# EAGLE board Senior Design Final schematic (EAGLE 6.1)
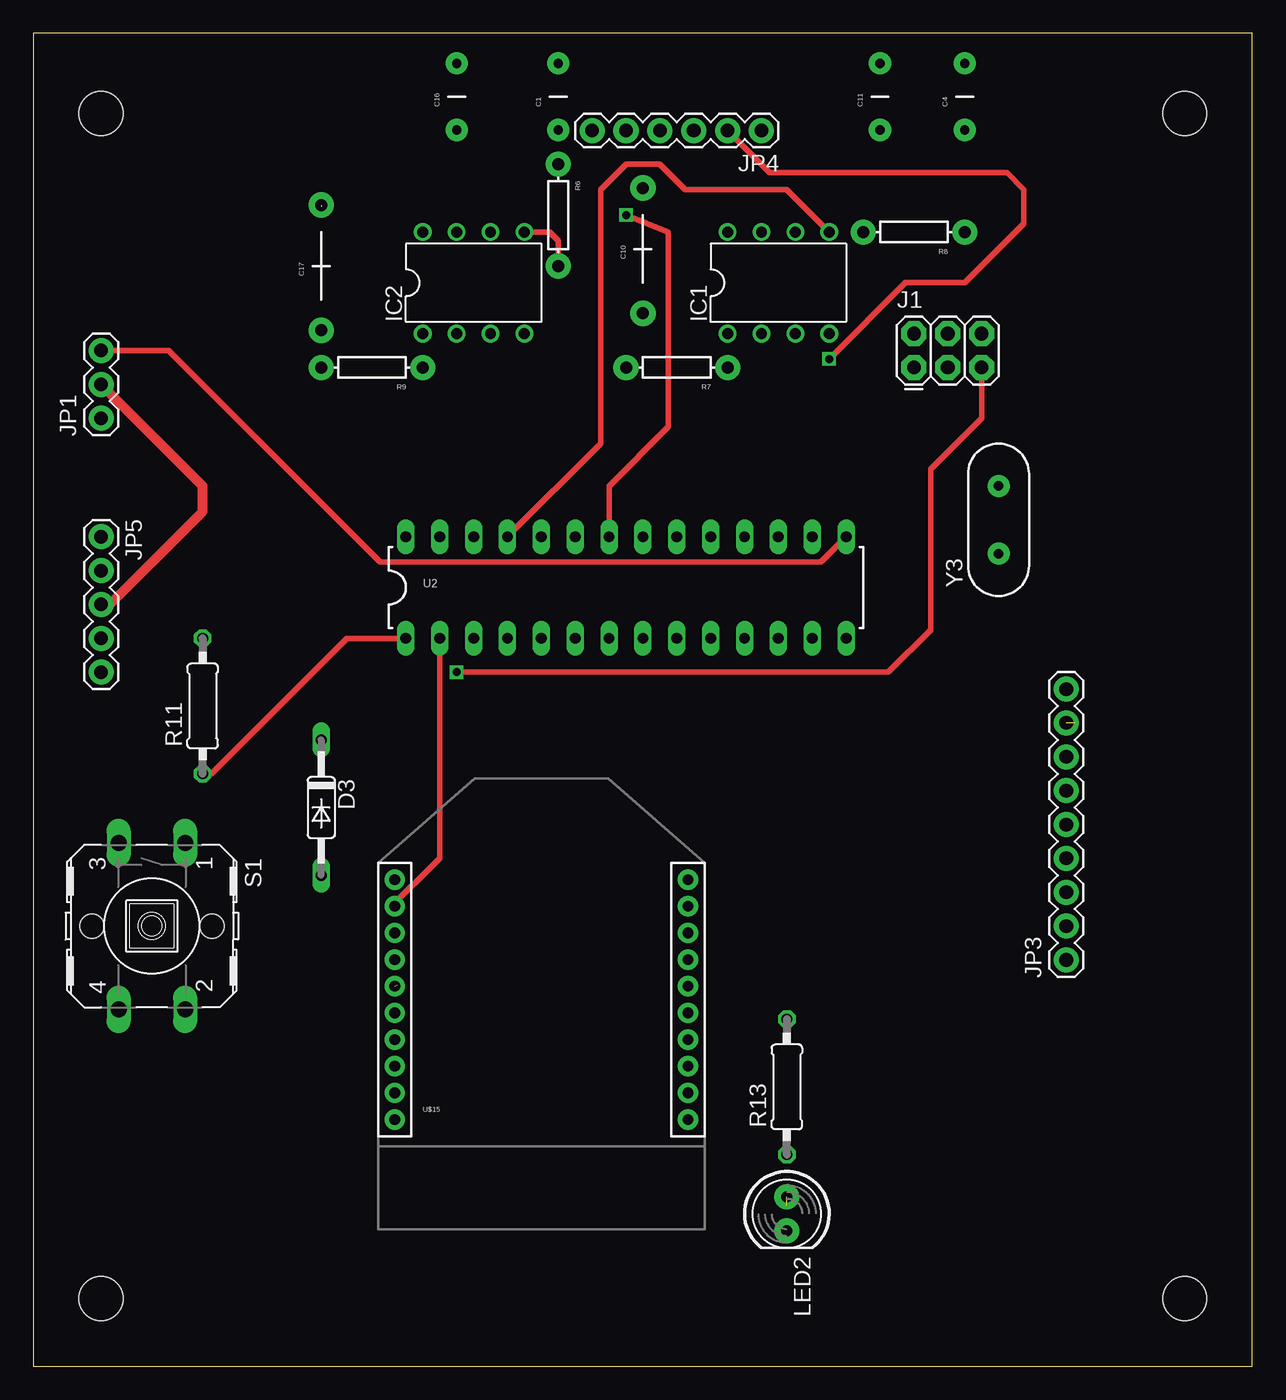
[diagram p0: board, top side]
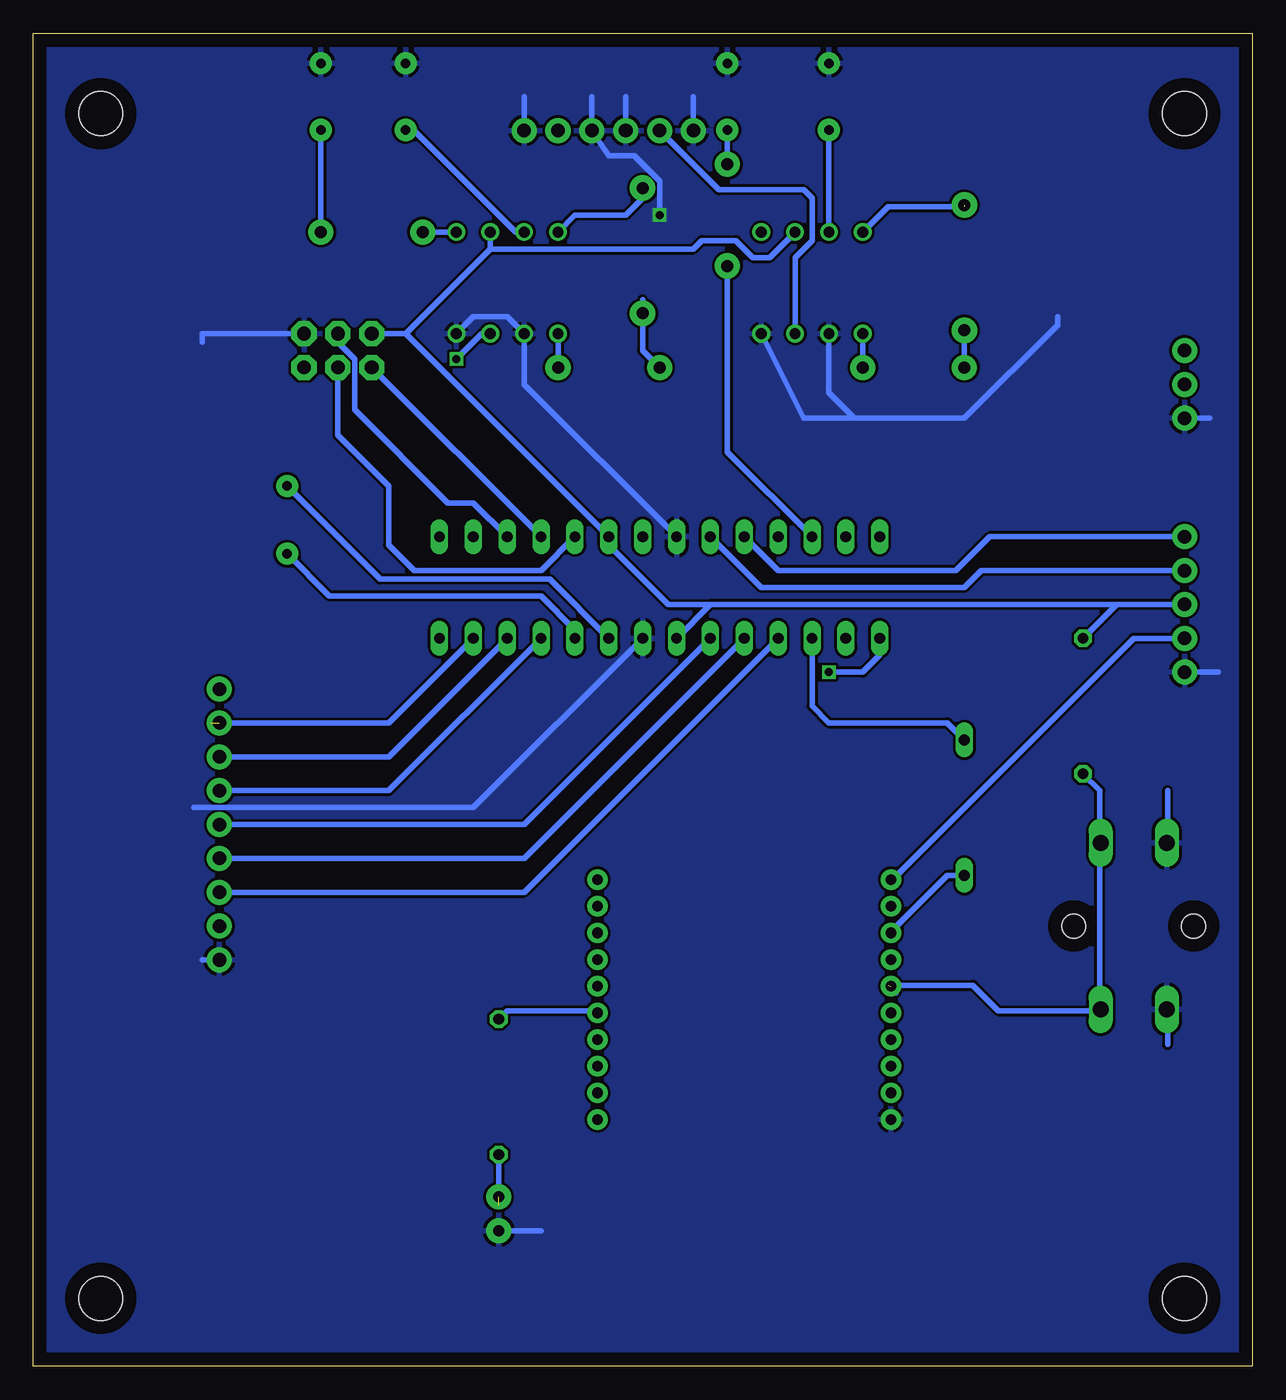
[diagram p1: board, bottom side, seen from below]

Size 91.42 x 100 mm. Coordinates in mm from the lower left corner, seen from the top.
Outline: 0,0 91.42,0 91.42,100 0,100 0,0
Copper layers (1*16): Top 0.035mm / dielectric 1.5mm / Bottom 0.035mm
Design rules: minimum track width 10mil, minimum drill 24mil, track to track 8mil, track to pad 8mil, pad to pad 8mil, via to via 8mil, smd to smd 8mil, copper to edge 40mil, drill to drill 8mil, minimum pad ring 10mil, minimum via ring 8mil, stop-mask expansion 4mil, vias tented up to drill 0mil, thermal gap 10mil

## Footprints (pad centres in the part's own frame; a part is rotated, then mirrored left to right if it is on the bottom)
CAP-PTH-5MM = drill 0.7 pad 1.651: 1 -2.5,0; 2 2.5,0
CAP-PTH-LARGE = drill 0.9 pad 1.905: 1 -4.826,0; 2 4.572,0
DO35-10 = drill 0.813 long: A 5.08,0; C -5.08,0
DIL08 = drill 0.813 pad 1.27: 1 -3.81,-3.81; 2 -1.27,-3.81; 3 1.27,-3.81; 4 3.81,-3.81; 5 3.81,3.81; 6 1.27,3.81; 7 -1.27,3.81; 8 -3.81,3.81
2X3 = drill 1.016 pad 1.88 octagon: 1 0,0; 2 0,2.54; 3 2.54,0; 4 2.54,2.54; 5 5.08,0; 6 5.08,2.54
1X03 = drill 1.016 pad 1.88: 1 0,0; 2 2.54,0; 3 5.08,0
1X09 = drill 1.016 pad 1.88: 1 0,0; 2 2.54,0; 3 5.08,0; 4 7.62,0; 5 10.16,0; 6 12.7,0; 7 15.24,0; 8 17.78,0; 9 20.32,0
1X06 = drill 1.016 pad 1.88: 1 0,0; 2 2.54,0; 3 5.08,0; 4 7.62,0; 5 10.16,0; 6 12.7,0
1X05 = drill 1.016 pad 1.88: 1 0,0; 2 2.54,0; 3 5.08,0; 4 7.62,0; 5 10.16,0
LED5MM = drill 0.813 pad 1.88: A -1.27,0; K 1.27,0
AXIAL-0.3 = drill 0.9 pad 1.88: P$1 -3.81,0; P$2 3.81,0
0207/10 = drill 0.813 octagon: 1 -5.08,0; 2 5.08,0
B3F-40XX = drill 1.194 long: 1 -6.248,2.489; 2 6.248,2.489; 3 -6.248,-2.489; 4 6.248,-2.489 | hole 1.803: 0,-4.496; 0,4.496
STAND-OFF = hole 3.302: 0,0
DIL28-3 = drill 0.813 long: 1 -16.51,-3.81; 2 -13.97,-3.81; 3 -11.43,-3.81; 4 -8.89,-3.81; 5 -6.35,-3.81; 6 -3.81,-3.81; 7 -1.27,-3.81; 8 1.27,-3.81; 9 3.81,-3.81; 10 6.35,-3.81; 11 8.89,-3.81; 12 11.43,-3.81; 13 13.97,-3.81; 14 16.51,-3.81; 15 16.51,3.81; 16 13.97,3.81; 17 11.43,3.81; 18 8.89,3.81; 19 6.35,3.81; 20 3.81,3.81; 21 1.27,3.81; 22 -1.27,3.81; 23 -3.81,3.81; 24 -6.35,3.81; 25 -8.89,3.81; 26 -11.43,3.81; 27 -13.97,3.81; 28 -16.51,3.81
XBEE-1 = drill 0.8 pad 1.524: 1 -11,20; 2 -11,18; 3 -11,16; 4 -11,14; 5 -11,12; 6 -11,10; 7 -11,8; 8 -11,6; 9 -11,4; 10 -11,2; 11 11,2; 12 11,4; 13 11,6; 14 11,8; 15 11,10; 16 11,12; 17 11,14; 18 11,16; 19 11,18; 20 11,20
HC49US = drill 0.7 pad 1.651: 1 -2.54,0; 2 2.54,0

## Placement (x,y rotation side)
C1  [CAP-PTH-5MM]  39.37,95.25 90 top
C4  [CAP-PTH-5MM]  69.85,95.25 90 top
C10  [CAP-PTH-LARGE]  45.72,83.82 90 top
C11  [CAP-PTH-5MM]  63.5,95.25 90 top
C16  [CAP-PTH-5MM]  31.75,95.25 90 top
C17  [CAP-PTH-LARGE]  21.59,82.55 90 top
D3  1N4446  [DO35-10]  21.59,41.91 270 top
IC1  LM386N-4  [DIL08]  55.88,81.28 0 top
IC2  LM386N-4  [DIL08]  33.02,81.28 0 top
J1  AVR_SPI_PRG_6PTH  [2X3]  66.04,74.93 0 top
JP1  [1X03]  5.08,71.12 90 top
JP3  M09  [1X09]  77.47,30.48 90 top
JP4  [1X06]  54.61,92.71 180 top
JP5  [1X05]  5.08,62.23 270 top
LED2  [LED5MM]  56.52,11.43 270 top
R6  [AXIAL-0.3]  39.37,86.36 270 top
R7  [AXIAL-0.3]  48.26,74.93 180 top
R8  [AXIAL-0.3]  66.04,85.09 180 top
R9  [AXIAL-0.3]  25.4,74.93 180 top
R11  [0207/10]  12.7,49.53 90 top
R13  [0207/10]  56.52,20.95 90 top
S1  [B3F-40XX]  8.89,33.02 270 top
STANDOFF  [STAND-OFF]  5.08,93.98 0 top
U2  ATMEGA328P_PDIP  [DIL28-3]  44.45,58.42 0 top
U$2  [STAND-OFF]  5.08,5.08 0 top
U$3  [STAND-OFF]  86.36,5.08 0 top
U$4  [STAND-OFF]  86.36,93.98 0 top
U$15  XBEE-1B1  [XBEE-1]  38.1,16.51 0 top
Y3  [HC49US]  72.39,63.5 90 top

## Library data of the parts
C1 C4 C10 C11 C16 C17 R6-R9 = SparkFun-Passives
D3 = diode
IC1 IC2 = linear
J1 JP1 JP3-JP5 = SparkFun-Connectors
LED2 = SparkFun-LED
R11 R13 = rcl
S1 = switch-omron; MF: OMRON COMPONENTS USA; MPN: B3F-4000; OC_FARNELL: 176434; OC_NEWARK: 36K3105
STANDOFF U$2-U$4 = SparkFun-Electromechanical
U2 = SparkFun-DigitalIC
U$15 = SparkFun-RF
Y3 = SparkFun-FreqCtrl

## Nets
3.3V: JP5.4 U$15.1
5V: IC1.6 IC2.6 J1.2 JP1.2 JP5.3 R11.2 U2.7 U2.20
AUDIO_DETECT: IC1.5 R8.P$2 U2.25
AUDIO_DETECT_2: IC2.5 R6.P$2 U2.26
AUDIO_IN_1: IC1.3 JP4.2
AUDIO_IN_2: IC2.3 JP4.5
GAIN_1: IC1.1 R7.P$1
GAIN_1_2: IC2.1 R9.P$1
GAIN_8: C10.2 IC1.8
GAIN_8_2: C17.2 IC2.8
GND: C1.2 C4.2 C11.2 C16.2 IC1.2 IC1.4 IC2.2 IC2.4 J1.6 JP1.1 JP3.1 JP4.1 JP4.3 JP4.4 JP4.6 JP5.5 LED2.K S1.3 S1.4 U2.8 U2.22 U$15.10
I_SENSE: JP5.2 U2.23
MC_1: JP3.3 U2.4
MC_2: JP3.4 U2.5
MC_3: JP3.5 U2.6
MC_4: JP3.6 U2.11
MC_5: JP3.7 U2.12
MC_6: JP3.8 U2.13
MISO_1: J1.1 U2.18
MOSI_1: J1.4 U2.17
N$1: R13.2
N$2: D3.C U2.3
N$3: D3.A U$15.3
N$4: U2.2 U$15.2
N$12: C11.1 IC1.7
N$13: C10.1 R7.P$2
N$16: U2.10 Y3.1
N$17: U2.9 Y3.2
N$20: LED2.A R13.1
N$24: C16.1 IC2.7
N$27: C1.1 R6.P$1
N$28: C4.1 R8.P$1
N$29: C17.1 R9.P$2
PAN_SIGNAL: JP1.3 U2.15
RESET_1: J1.5 R11.1 S1.1 S1.2 U2.1 U$15.5
S$1: U$15.15
SCK_1: J1.3 U2.19
V_SENSE: JP5.1 U2.24

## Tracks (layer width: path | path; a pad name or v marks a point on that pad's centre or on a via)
3.3V
  Bottom 0.254: 26.67,36.83 U$15.1
  Bottom 0.406: JP5.4 8.89,54.61 26.67,36.83 27.3,36.2
5V
  Top 0.762: JP5.3 5.71,57.15 12.7,64.14 12.7,66.04 JP1.2
  Bottom 0.406: 40.64,57.15 JP5.3 10.16,57.15 R11.2 | 40.64,57.15 U2.7 | 40.64,57.15 43.81,57.15 48.26,61.59 U2.20 63.5,77.47 | 63.5,77.47 J1.2 | 63.5,77.47 57.15,83.82 | 57.15,83.82 IC1.6 | 57.15,83.82 41.91,83.82 41.27,84.45 38.73,84.45 37.47,83.19 36.2,83.19 IC2.6
AUDIO_DETECT
  Top 0.406: IC1.5 56.52,88.27 48.9,88.27 46.99,90.17 44.45,90.17 42.55,88.27 42.55,69.22 U2.25
  Bottom 0.406: R8.P$2 IC1.5
AUDIO_DETECT_2
  Top 0.406: R6.P$2 39.37,84.45 38.73,85.09 IC2.5
  Bottom 0.406: R6.P$2 39.37,68.58 U2.26
AUDIO_IN_1  (via drill 0.6)
  Top 0.406: v59.69,75.56 65.41,81.28 69.85,81.28 74.3,85.72 74.3,88.27 73.03,89.53 55.24,89.53 JP4.2
  Bottom 0.406: IC1.3 57.78,77.47 v59.69,75.56
AUDIO_IN_2
  Bottom 0.406: IC2.3 34.29,83.19 33.02,84.45 33.02,87.63 33.66,88.27 40.01,88.27 JP4.5
GAIN_1
  Bottom 0.406: IC1.1 R7.P$1
GAIN_1_2
  Bottom 0.406: IC2.1 R9.P$1
GAIN_8
  Bottom 0.406: 45.72,88.9 C10.2 45.72,87.63 46.99,86.36 50.8,86.36 IC1.8
GAIN_8_2  (1 unrouted)
  Bottom 0.254: 21.59,86.36 C17.2
  Bottom 0.406: IC2.8 27.3,87 21.59,87
GND  (via drill 0.6)
  Top 0.406: U2.22 43.18,66.04 47.62,70.48 47.62,85.09 v44.45,86.36
  Bottom 0.406: LED2.K 53.34,10.16 | JP3.1 78.74,30.48 | JP5.5 2.54,52.07 | U2.8 58.42,41.91 79.38,41.91 | JP4.6 41.91,95.25 | JP4.4 46.99,95.25 | 49.53,95.25 JP4.3 48.26,90.81 46.35,90.81 44.45,88.9 v44.45,86.36 | JP4.1 54.61,95.25 | IC2.2 31.75,73.03 29.84,71.12 | 29.84,71.12 21.59,71.12 14.61,78.11 14.61,78.74 | IC2.4 33.66,71.12 29.84,71.12 | U2.22 54.61,73.66 IC1.2 55.88,78.74 58.42,78.74 IC1.4 | JP1.1 3.17,71.12 | J1.6 78.74,77.47 78.74,76.83
  pour Bottom: 0,53.34 8.26,53.34 8.26,19.68 45.72,19.68 45.72,12.7 45.72,10.79 75.56,10.79 75.56,31.75 78.74,31.75 78.74,45.72 91.44,45.72 91.44,0 0,0
  pour Bottom: 0,53.34 3.81,53.34 3.81,78.11 20.32,78.11 20.32,94.61 78.74,94.61 78.74,45.72 91.44,45.72 91.44,100.33 0,100.33
  pour Bottom: -1.91,101.6 -1.91,-1.27 94.61,-1.27 94.61,101.6
I_SENSE
  Bottom 0.406: JP5.2 20.32,59.69 21.59,58.42 36.83,58.42 U2.23
MC_1
  Bottom 0.406: JP3.3 54.61,35.56 U2.4
MC_2
  Bottom 0.406: JP3.4 54.61,38.1 U2.5
MC_3
  Bottom 0.406: JP3.5 54.61,40.64 U2.6
MC_4
  Bottom 0.406: JP3.6 64.77,43.18 U2.11
MC_5
  Bottom 0.406: JP3.7 64.77,45.72 U2.12
MC_6  (1 unrouted)
  Bottom 0.406: 78.11,48.26 64.77,48.26 U2.13
MISO_1
  Bottom 0.406: J1.1 U2.18
MOSI_1
  Bottom 0.406: J1.4 68.58,76.83 67.31,75.56 67.31,71.75 60.33,64.77 58.42,64.77 U2.17
N$1
  Bottom 0.406: 48.9,26.67 55.88,26.67 R13.2
N$2
  Bottom 0.406: U2.3 33.02,49.53 31.75,48.26 22.86,48.26 D3.C
N$3
  Bottom 0.254: 26.67,33.02 U$15.3
  Bottom 0.406: 27.3,32.38 26.67,33.02 22.86,36.83 D3.A
N$4
  Top 0.254: 26.67,34.29 U$15.2
  Top 0.406: U2.2 30.48,38.1 26.67,34.29
N$7
  Bottom 0.406: 6.35,39.37 6.35,43.18
N$8
  Bottom 0.406: 6.35,26.67 6.35,24.13
N$12
  Bottom 0.254: 63.5,92.71 C11.1
  Bottom 0.406: IC1.7 55.24,85.09 62.87,92.71 63.5,92.71 64.14,92.71
N$13
  Bottom 0.406: R7.P$2 45.72,76.2 C10.1 45.72,80.01
N$16
  Bottom 0.406: U2.10 50.8,55.24 53.34,57.78 69.22,57.78 Y3.1
N$17
  Bottom 0.406: U2.9 52.7,59.05 65.41,59.05 Y3.2
N$20  (1 unrouted)
  Bottom 0.406: R13.1 56.52,12.06
N$24
  Bottom 0.254: 31.75,92.71 C16.1
  Bottom 0.406: IC2.7 31.75,92.71
N$27
  Bottom 0.254: 39.37,92.71 C1.1
  Bottom 0.406: R6.P$1 39.37,92.71
N$28
  Bottom 0.254: 69.85,92.71 C4.1
  Bottom 0.406: 69.85,92.71 R8.P$1
N$29
  Bottom 0.406: 21.59,78.11 C17.1 R9.P$2
PAN_SIGNAL
  Top 0.406: U2.15 59.05,60.33 26.04,60.33 10.16,76.2 JP1.3
RESET_1  (via drill 0.6)  (1 unrouted)
  Top 0.406: R11.1 13.34,44.45 23.5,54.61 U2.1 | v31.75,52.07 64.14,52.07 67.31,55.24 67.31,67.31 71.12,71.12 J1.5
  Bottom 0.254: 11.43,27.94 S1.2 | 11.43,39.37 S1.1 | 26.67,27.94 U$15.5
  Bottom 0.406: 27.3,28.57 20.95,28.57 19.05,26.67 11.43,26.67 11.43,27.94 11.43,39.37 11.43,43.18 R11.1 | U2.1 27.94,53.34 29.21,52.07 v31.75,52.07
SCK_1
  Bottom 0.406: J1.3 68.58,69.85 64.77,66.04 64.77,61.59 62.87,59.69 53.34,59.69 U2.19
V_SENSE
  Bottom 0.406: JP5.1 19.68,62.23 22.23,59.69 35.56,59.69 U2.24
